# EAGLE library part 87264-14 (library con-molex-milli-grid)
RECEPTACAL
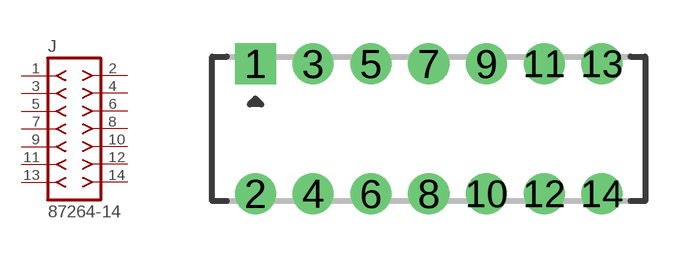
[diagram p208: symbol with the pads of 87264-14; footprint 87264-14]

Designator prefix J

## 87264-14  [87264-14]
1  1  pas
2  2  pas
3  3  pas
4  4  pas
5  5  pas
6  6  pas
7  7  pas
8  8  pas
9  9  pas
10  10  pas
11  11  pas
12  12  pas
13  13  pas
14  14  pas

## Footprint 87264-14 (pad centres in mm)
RECEPTACAL Dual Row, Side Entry
drill 0.914 square: 1 -6,2.25
drill 0.914: 2 -6,-2.25; 3 -4,2.25; 4 -4,-2.25; 5 -2,2.25; 6 -2,-2.25; 7 0,2.25; 8 0,-2.25; 9 2,2.25; 10 2,-2.25; 11 4,2.25; 12 4,-2.25; 13 6,2.25; 14 6,-2.25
